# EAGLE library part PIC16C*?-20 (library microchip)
MICROCONTROLLER Pin compatible devices PIC16C5X family: EPROM/ROM-based PIC16C55X family: EPROM-based PIC16C6X family PIC16CE62X family: analog comparators/EEPROM data memory PIC16C7X family: A/D converter PIC16C71X family: A/D converter Pin compatible devices: PIC16C154, PIC16CR154, PIC16C156, PIC16CR156, PIC16C158 PIC16CR158, PIC16C52, PIC16C54, PIC16C54A, PIC16CR54A PIC16C56, PIC16C58A, PIC16CR58A, PIC16C61, PIC16C554 PIC16C556, PIC16C558, PIC16C620, PIC16C621, PIC16C622 PIC16C641, PIC16C642, PIC16C661, PIC16C662, PIC16C71 PIC16C710, PIC16C711, PIC16C715, PIC126F83, PIC16CR83 PIC16F84A, PIC16CR84
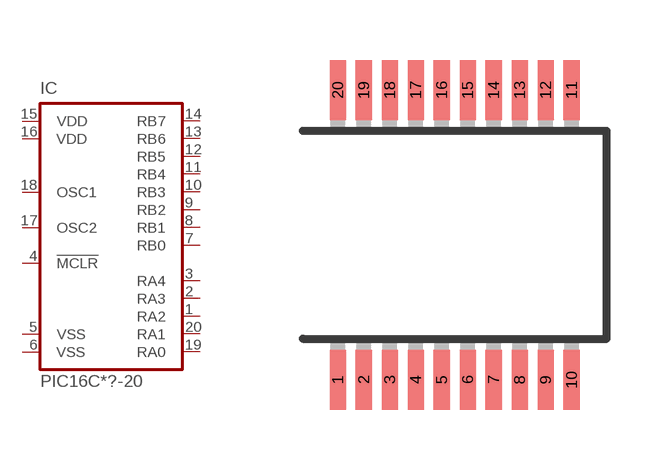
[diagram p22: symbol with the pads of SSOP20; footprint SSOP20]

Designator prefix IC

## PIC16C154SS-20 (OC_FARNELL: unknown; OC_NEWARK: unknown), PIC16C156SS-20 (OC_FARNELL: unknown; OC_NEWARK: unknown), PIC16C158SS-20 (OC_FARNELL: unknown; OC_NEWARK: unknown), PIC16C54SS-20 (MF: MICROCHIP; MPN: PIC16C54-RCI/SS; OC_FARNELL: unknown; OC_NEWARK: 23C3206), PIC16C54ASS-20 (OC_FARNELL: unknown; OC_NEWARK: unknown), PIC16C554SS-20 (OC_FARNELL: unknown; OC_NEWARK: unknown), PIC16C556SS-20 (OC_FARNELL: unknown; OC_NEWARK: unknown), PIC16C558SS-20 (MF: MICROCHIP; MPN: PIC16C558-20I/SS; OC_FARNELL: unknown; OC_NEWARK: 23C3497), PIC16C56SS-20 (MF: MICROCHIP; MPN: PIC16C56-HSI/SS; OC_FARNELL: 116506; OC_NEWARK: 23C3519), PIC16C58ASS-20 (MF: MICROCHIP; MPN: PIC16C58B-04/SS; OC_FARNELL: unknown; OC_NEWARK: 23C3738), PIC16C620SS-20 (MF: MICROCHIP; MPN: PIC16C620A-04/SS; OC_FARNELL: unknown; OC_NEWARK: 23C3858), PIC16C621SS-20 (MF: MICROCHIP; MPN: PIC16C621-20I/SS; OC_FARNELL: unknown; OC_NEWARK: 23C3915), PIC16C622SS-20 (MF: MICROCHIP; MPN: PIC16C622A-04/SS; OC_FARNELL: unknown; OC_NEWARK: 23C3980), PIC16C710SS-20 (OC_FARNELL: unknown; OC_NEWARK: unknown), PIC16C711SS-20 (MF: MICROCHIP; MPN: PIC16C711-04/SS; OC_FARNELL: unknown; OC_NEWARK: 23C4469), PIC16C715SS-20 (MF: MICROCHIP; MPN: PIC16C715-04/SS; OC_FARNELL: unknown; OC_NEWARK: 23C4525), PIC16CR154SS-20 (OC_FARNELL: unknown; OC_NEWARK: unknown), PIC16CR156SS-20 (OC_FARNELL: unknown; OC_NEWARK: unknown), PIC16CR158SS-20 (OC_FARNELL: unknown; OC_NEWARK: unknown), PIC16CR54ASS-20 (OC_FARNELL: unknown; OC_NEWARK: unknown), PIC16CR58ASS-20 (OC_FARNELL: unknown; OC_NEWARK: unknown)  [SSOP20]
1  RA2
2  RA3
3  RA4
4  !MCLR  in
5  VSS  pwr
6  VSS  pwr
7  RB0
8  RB1
9  RB2
10  RB3
11  RB4
12  RB5
13  RB6
14  RB7
15  VDD  pwr
16  VDD  pwr
17  OSC2  out
18  OSC1  in
19  RA0
20  RA1

## Footprint SSOP20 (pad centres in mm)
Shrink Small Outline Package package type SS
smd 0.4 x 1.5: 1 -2.925,-3.625; 2 -2.275,-3.625; 3 -1.625,-3.625; 4 -0.975,-3.625; 5 -0.325,-3.625; 6 0.325,-3.625; 7 0.975,-3.625; 8 1.625,-3.625; 9 2.275,-3.625; 10 2.925,-3.625; 11 2.925,3.625; 12 2.275,3.625; 13 1.625,3.625; 14 0.975,3.625; 15 0.325,3.625; 16 -0.325,3.625; 17 -0.975,3.625; 18 -1.625,3.625; 19 -2.275,3.625; 20 -2.925,3.625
